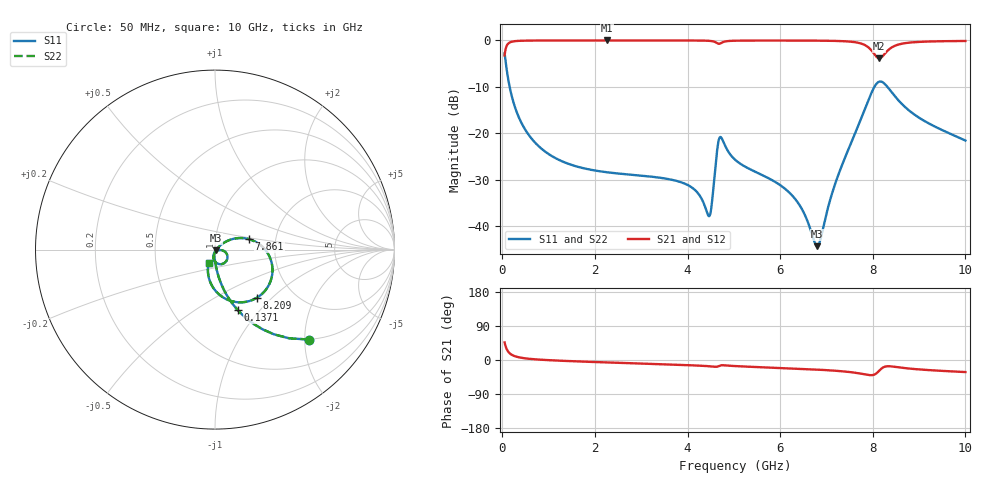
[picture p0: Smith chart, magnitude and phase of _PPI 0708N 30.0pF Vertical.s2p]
! S-Parameter data specifications (vertical orientation):
! Substrate: 40-mil Rogers 3003C, Substrate thickness, H=1.016mm, Dielectric constant, Er=3, Conductor thickness, T_mtl=0.043mm, Loss Tangent, Tand=0.003
! PCB Mounting Pad Footprint: Pad width, PadW=2.54mm , Pad length, PadL=0.51mm , Pad gap, PadG (edge-to-edge)=0.71mm , Reference planes=1.73mm apart
! Created Tue Jan 16 08:53:00 2018
# GHz S MA R 50
! 2 Port Network Data from SP1.SP block
! freq  magS11  angS11  magS21  angS21  magS12  angS12  magS22  angS22
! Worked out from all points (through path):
!   801 points, 50 MHz to 10 GHz, reference 50 ohm
!   highest |S21| = -0.01 dB at 2.264 GHz (marker M1); lowest = -3.9 dB at 8.134 GHz (marker M2)
!   group delay of S21, straight-line fit = 10.6 ps
!   lowest |S11| = -44.3 dB at 6.804 GHz (marker M3), VSWR 1.01, Z = 50.5 - j0.336 ohm
!   |S11| at or under -10 dB: 158.5 MHz to 8.036 GHz (7.877 GHz wide, 192 % of centre); 8.315 GHz to end of sweep
!   |S22| runs from -44.3 to -2.8 dB; largest |S21 - S12| = 0
!   S11 on the Smith chart (normalised r, x): 50 MHz: 0.99, -2.10; 137.1 MHz: 0.99, -0.77; 7.861 GHz: 1.46, +0.18; 8.209 GHz: 1.32, -0.81; 10 GHz: 0.92, -0.14
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0.05  0.7251 -43.7  0.6884 46.3  0.6884 46.3  0.7251 -43.7
0.1370625  0.3593 -69.4  0.933 20.5  0.933 20.5  0.3593 -69.4
0.3360625  0.1571 -82.2  0.9873 7.8  0.9873 7.8  0.1571 -82.2
0.647  0.0857 -87.4  0.996 2.4  0.996 2.4  0.0857 -87.4
1.716625  0.04237 -93.5  0.9985 -4.1  0.9985 -4.1  0.04237 -93.5
2.263875  0.03793 -95.6  0.9986 -6.5  0.9986 -6.5  0.03793 -95.6
3.370812  0.03331 -99.4  0.9984 -10.9  0.9984 -10.9  0.03331 -99.4
4.092187  0.02601 -99.8  0.9975 -14.0  0.9975 -14.0  0.02601 -99.8
4.452875  0.01287 -60.6  0.9906 -16.3  0.9906 -16.3  0.01287 -60.6
4.515062  0.01589 -22.6  0.984 -17.0  0.984 -17.0  0.01589 -22.6
4.639437  0.06562 -17.3  0.9342 -17.6  0.9342 -17.6  0.06562 -17.3
4.701625  0.0909 -50.3  0.9244 -14.8  0.9244 -14.8  0.0909 -50.3
5.025  0.05189 -99.1  0.9922 -16.0  0.9922 -16.0  0.05189 -99.1
6.206563  0.0227 -103.9  0.9963 -22.0  0.9963 -22.0  0.0227 -103.9
6.691625  0.008016 -74.7  0.9945 -24.7  0.9945 -24.7  0.008016 -74.7
6.803562  0.006064 -33.3  0.9937 -25.4  0.9937 -25.4  0.006064 -33.3
7.214  0.03108 37.6  0.9867 -28.5  0.9867 -28.5  0.03108 37.6
7.86075  0.1994 16.8  0.873 -38.7  0.873 -38.7  0.1994 16.8
8.134375  0.3586 -32.5  0.6415 -28.9  0.6415 -28.9  0.3586 -32.5
8.209  0.3554 -49.0  0.6724 -20.7  0.6724 -20.7  0.3554 -49.0
8.345812  0.3028 -71.8  0.796 -16.5  0.796 -16.5  0.3028 -71.8
10  0.08333 -114.8  0.9859 -31.8  0.9859 -31.8  0.08333 -114.8
